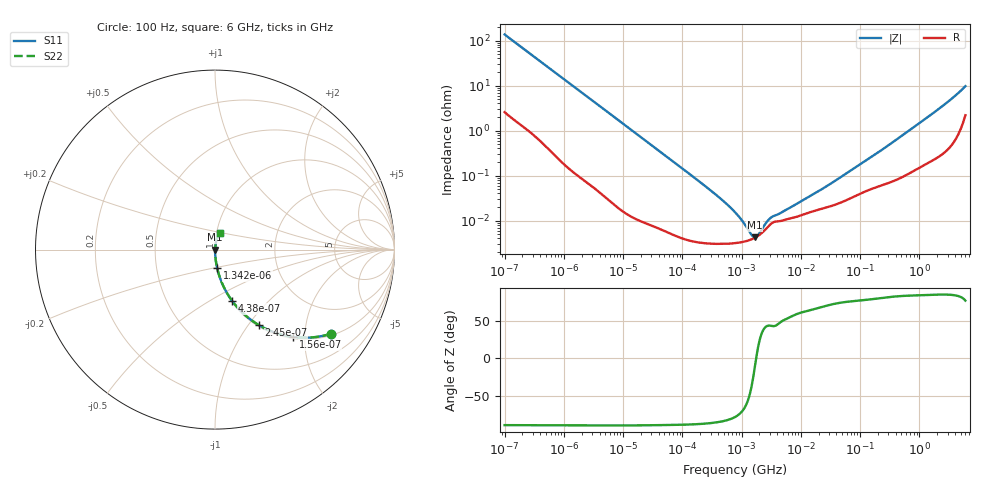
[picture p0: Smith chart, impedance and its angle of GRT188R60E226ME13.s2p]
!Murata Part Number: GRT188R60E226ME13
!These Parameters are Measured in Series Mode Connection
!Data Generated on Jun 19, 2026
!  o--ll--o
!Port1  Port2
!  o------o
!Operation Temp=25[degC], DC Bias Voltage=0[V]
!Freq. Start=100[Hz] Stop=6[GHz] 401[Steps]
# Hz S RI R 50
!Freq.(Hz) S11(Real) S11(Imag) S21(Real) S21(Imag) S12(Real) S12(Imag) S22(Real) S22(Imag)
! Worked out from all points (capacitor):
!   401 points, 100 Hz to 6 GHz, reference 50 ohm
!   read as one part in series: C = 11.6 uF near 109 Hz
!   lowest |Z| = 4.24 mohm at 1.658 MHz (marker M1)
!   series resonance near 1.762 MHz, so ESL is about 700 pH
!   S11 on the Smith chart (normalised r, x): 100 Hz: 1.05, -2.72; 156 Hz: 1.03, -1.75; 245 Hz: 1.02, -1.12; 438 Hz: 1.01, -0.63; 1.342 kHz: 1.00, -0.21; 6 GHz: 1.04, +0.19
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100  0.6473 -0.4685  0.3527 0.4685  0.3527 0.4685  0.6473 -0.4685
156  0.4347 -0.4867  0.5653 0.4867  0.5653 0.4867  0.4347 -0.4867
245  0.244 -0.4206  0.756 0.4206  0.756 0.4206  0.244 -0.4206
320  0.1611 -0.3589  0.8389 0.3589  0.8389 0.3589  0.1611 -0.3589
438  0.0948 -0.2849  0.9052 0.2849  0.9052 0.2849  0.0948 -0.2849
717  0.0388 -0.1862  0.9612 0.1862  0.9612 0.1862  0.0388 -0.1862
1342  0.012 -0.1028  0.988 0.1028  0.988 0.1028  0.012 -0.1028
2008  0.00569 -0.0694  0.9943 0.0694  0.9943 0.0694  0.00569 -0.0694
6433  0.000731 -0.022  0.9993 0.022  0.9993 0.022  0.000731 -0.022
40335  7.87e-05 -0.00354  0.9999 0.00354  0.9999 0.00354  7.87e-05 -0.00354
316350  3.08e-05 -0.000442  1 0.000442  1 0.000442  3.08e-05 -0.000442
541393  3.06e-05 -0.000242  1 0.000242  1 0.000242  3.06e-05 -0.000242
774597  3.15e-05 -0.00015  1 0.00015  1 0.00015  3.15e-05 -0.00015
968953  3.29e-05 -0.000104  1 0.000104  1 0.000104  3.29e-05 -0.000104
1059725  3.36e-05 -8.7e-05  1 8.7e-05  1 8.7e-05  3.36e-05 -8.7e-05
1658239  4.12e-05 -9.9e-06  1 9.9e-06  1 9.9e-06  4.12e-05 -9.9e-06
2713602  7e-05 6.6e-05  0.9999 -6.6e-05  0.9999 -6.6e-05  7e-05 6.6e-05
1.555665e7  0.000159 0.000339  0.9998 -0.000339  0.9998 -0.000339  0.000159 0.000339
3.64232e7  0.000221 0.000705  0.9998 -0.000705  0.9998 -0.000705  0.000221 0.000705
3.124326e8  0.000717 0.00481  0.9993 -0.00481  0.9993 -0.00481  0.000717 0.00481
2.142435e9  0.00353 0.0301  0.9965 -0.0301  0.9965 -0.0301  0.00353 0.0301
6e9  0.0297 0.0898  0.9703 -0.0898  0.9703 -0.0898  0.0297 0.0898
